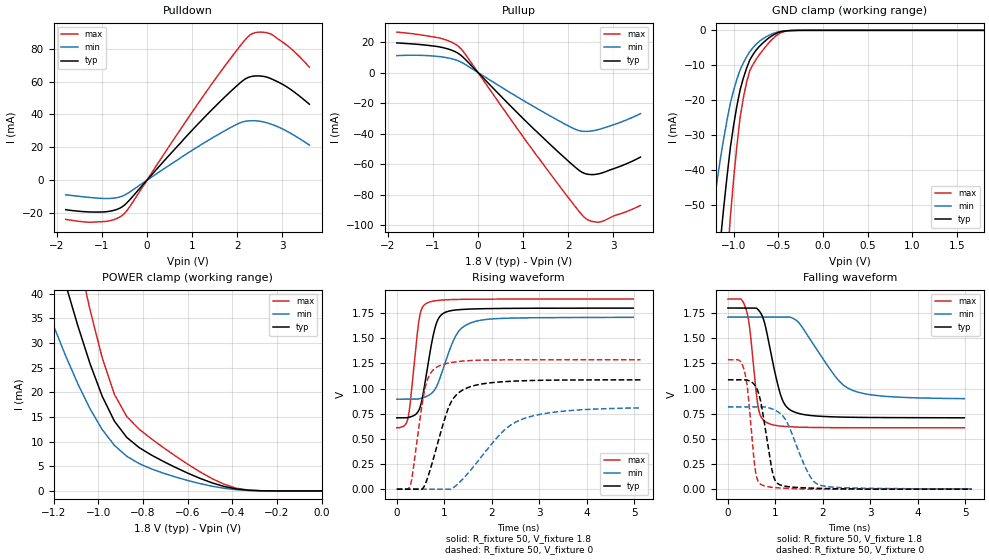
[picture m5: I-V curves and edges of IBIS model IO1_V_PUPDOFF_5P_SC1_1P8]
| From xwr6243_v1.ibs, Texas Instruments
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|   Model Cell IO1_V_PUPDOFF_5P_SC1_1P8
|IO1_V_PUPDOFF_5P_SC1_1P8
[Model]   IO1_V_PUPDOFF_5P_SC1_1P8
Model_type   I/O
Polarity   Non-Inverting
Enable   Active-Low
Vinl =  0.63
Vinh =  1.17
Cref =  15pF
Rref =  100.0000M
Vref =  0V
Vmeas =  0.9
|   typ   min   max
C_comp   2.233931p   2.204415p   2.290246p
[Model Spec]
Vinl   0.63   0.5985   0.6615
Vinh   1.17   1.1115   1.2285
[Temperature Range]   25   125   -40
[Voltage Range]   1.8   1.71   1.89
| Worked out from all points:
|   slope of the pulldown table from 0 to 0.27 V, typ, clamps not added: 32.2 ohm
|   slope of the pullup table from 0 to 0.27 V, typ, clamps not added: 32.6 ohm
|   GND clamp passes 1 mA (typ) near -0.53 V on its own axis
|   POWER clamp passes 1 mA (typ) near -0.44 V on its own axis
|   rising waveform, R_fixture 50, V_fixture 1.8: 20-80 % time 246ps typ, 396ps min, 169ps max; typ from 0.709 V to 1.8 V
|   rising waveform, R_fixture 50, V_fixture 0: 20-80 % time 429ps typ, 920ps min, 245ps max; typ from 0 V to 1.09 V
|   falling waveform, R_fixture 50, V_fixture 1.8: 20-80 % time 308ps typ, 718ps min, 171ps max; typ from 1.8 V to 0.709 V
|   falling waveform, R_fixture 50, V_fixture 0: 20-80 % time 226ps typ, 430ps min, 154ps max; typ from 1.09 V to 0 V
| Where Nom  PVT is Nominal Process, 1.8V, 25C
|   Fast PVT is Strong Process,  1.89V, -40C
|   Slow PVT is Weak Process,   1.71V, 125C
[POWER_clamp]
|   voltage   I(typ)   I(min)   I(max)
-1.8V     158.8mA    112.5mA    219.7mA
-1.255V   59.93mA    39.99mA    84.86mA
-1.127V   39.08mA    25.5mA     55.75mA
-1.055V   28.36mA    18.34mA    40.41mA
-981.8mV  19.18mA    12.43mA    26.98mA
-927.3mV  14.16mA    9.239mA    19.58mA
-872.7mV  10.89mA    7.049mA    15.14mA
-818.2mV  8.843mA    5.579mA    12.59mA
-600mV    3.63mA     2.128mA    5.45mA
-436.4mV  903.9uA    539uA      1.358mA
-327.3mV  138.2uA    94.87uA    160.3uA
0V        19.3nA     133.7nA    230.3nA
[Pulldown]
|   voltage   I(typ)   I(min)   I(max)
-1.8V     -17.92mA   -8.85mA    -23.8mA
-1.309V   -19.26mA   -10.37mA   -25.5mA
-927.3mV  -19.22mA   -11.12mA   -25.08mA
-654.5mV  -17.65mA   -10.56mA   -23.13mA
-490.9mV  -14.97mA   -8.985mA   -20.05mA
1.364V    40.78mA    24.32mA    55.7mA
2.073V    59.41mA    35mA       81.91mA
2.291V    62.96mA    36.2mA     88.48mA
2.509V    63.41mA    35.84mA    90.12mA
2.782V    61.38mA    33.82mA    88.42mA
3.218V    54.59mA    28.02mA    79.45mA
3.6V      46.26mA    21.39mA    68.79mA
[Pullup]
|   voltage   I(typ)   I(min)   I(max)
-1.8V     19.42mA    11.07mA    26.5mA
-818.2mV  16.58mA    10.3mA     22.34mA
-545.5mV  14.19mA    8.748mA    19.29mA
-381.8mV  11.34mA    6.915mA    15.7mA
1.255V    -37.51mA   -22.64mA   -52.53mA
2.127V    -61.34mA   -36.82mA   -86.78mA
2.291V    -65.12mA   -38.38mA   -92.82mA
2.4V      -66.46mA   -38.59mA   -95.91mA
2.564V    -66.86mA   -38.08mA   -97.75mA
2.727V    -65.99mA   -36.9mA    -97.78mA
3.273V    -60.01mA   -31.26mA   -91.34mA
3.6V      -55.4mA    -26.98mA   -87.12mA
[GND_clamp]
|   voltage   I(typ)   I(min)   I(max)
-1.8V     -270.2mA   -170.2mA   -430.1mA
-1.255V   -91.66mA   -55.91mA   -148.4mA
-1.145V   -59.91mA   -36.45mA   -97.09mA
-1.109V   -50.48mA   -30.83mA   -81.55mA
-1.073V   -41.73mA   -25.65mA   -67.05mA
-1.036V   -33.66mA   -20.92mA   -53.59mA
-927.3mV  -17.07mA   -11.35mA   -25.04mA
-854.5mV  -10.86mA   -7.617mA   -14.91mA
-781.8mV  -6.919mA   -4.945mA   -9.771mA
-636.4mV  -2.823mA   -1.868mA   -4.529mA
-381.8mV  -84.73uA   -78.82uA   -126.1uA
1.8V      19.3nA     350.9nA    215.8nA
[Ramp]
| variable   typ   min   max
dV/dt_f 0.66170167/0.31099078n 0.49657778/0.73394202n 0.77361898/0.17271731n
dV/dt_r 0.65944933/0.43266271n 0.50305793/0.9625316n 0.77800654/0.24641056n
R_load = 50
[Rising Waveform]
R_fixture = 50
V_fixture = 1.8
V_fixture_min = 1.71
V_fixture_max = 1.89
|   time   V(typ)   V(min)   V(max)
0s        709.3mV    894.5mV    611.4mV
234.6ps   711.5mV    894.5mV    703.8mV
472.5ps   793.4mV    898.9mV    1.696V
530.6ps   889.7mV    906mV      1.8V
629.4ps   1.164V     923.1mV    1.849V
776.9ps   1.552V     975.4mV    1.871V
893ps     1.709V     1.085V     1.878V
1.246ns   1.782V     1.529V     1.886V
1.554ns   1.791V     1.653V     1.888V
4.974ns   1.8V       1.708V     1.89V
[Rising Waveform]
R_fixture = 50
V_fixture = 0
V_fixture_min = 0
V_fixture_max = 0
|   time   V(typ)   V(min)   V(max)
0s        0V         0V         0V
286.6ps   0V         0V         43.73mV
599.1ps   50.7mV     0V         1.014V
699.4ps   189mV      0V         1.144V
867.6ps   469.4mV    0V         1.22V
1.163ns   882.5mV    6.887mV    1.26V
1.567ns   1.022V     196.1mV    1.279V
2.232ns   1.068V     573.7mV    1.286V
2.671ns   1.078V     701.1mV    1.286V
5.128ns   1.087V     807.5mV    1.286V
[Falling Waveform]
R_fixture = 50
V_fixture = 1.8
V_fixture_min = 1.71
V_fixture_max = 1.89
|   time   V(typ)   V(min)   V(max)
0s        1.8V       1.71V      1.889V
275ps     1.8V       1.71V      1.889V
378.3ps   1.8V       1.71V      1.793V
458.3ps   1.8V       1.71V      1.601V
639.6ps   1.782V     1.71V      808.7mV
817.6ps   1.558V     1.71V      661.9mV
1.117ns   924.6mV    1.71V      626.1mV
1.374ns   771.3mV    1.697V     618.4mV
2.562ns   714.5mV    994.7mV    610.4mV
4.974ns   709mV      899.8mV    610mV
[Falling Waveform]
R_fixture = 50
V_fixture = 0
V_fixture_min = 0
V_fixture_max = 0
|   time   V(typ)   V(min)   V(max)
0s        1.087V     818.1mV    1.286V
342.4ps   1.087V     818.1mV    1.182V
418.5ps   1.082V     818.1mV    969.6mV
572.1ps   1.029V     818.1mV    202.3mV
701ps     843.3mV    818.1mV    45.39mV
938.3ps   167.4mV    795.8mV    17.73mV
1.101ns   42.19mV    751.8mV    11.59mV
1.704ns   11.22mV    148.3mV    0V
1.916ns   8.516mV    43.66mV    0V
5.128ns   0V         2.183mV    0V
